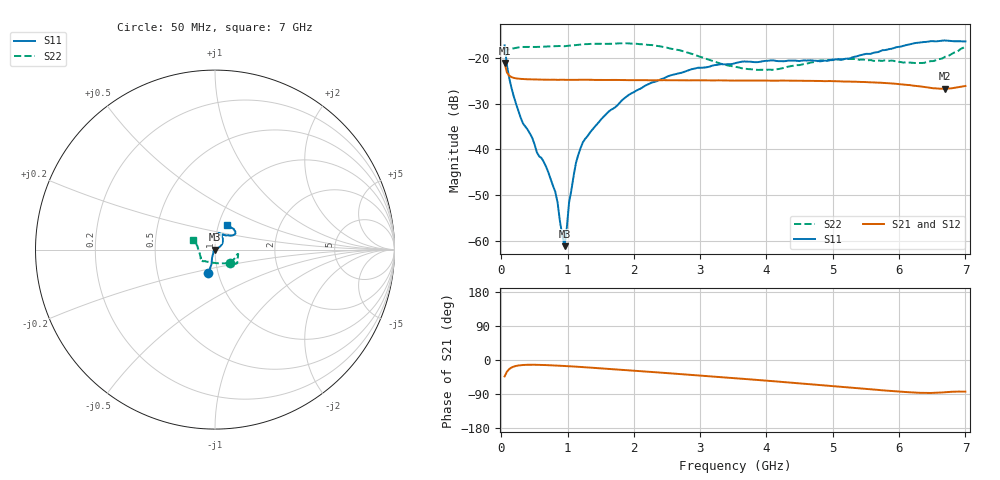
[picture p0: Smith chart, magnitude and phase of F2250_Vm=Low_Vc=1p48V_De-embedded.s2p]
! Integrated Device Technology
! Corporate Headquarters
! 6024 Silver Creek Valley Road
! San Jose, CA 95138  USA
! Phone:  1-408-284-8200
! Toll Free:  1-800-223-1366
! Webpage:  http://www.idt.com/
! Timing and RF Division
! 515 Groton Road, Suite 102
! Westford, MA 01886-6024
! Device:  F2250
! Description: Voltage Variable RF Attenuator
! Frequency:  50.0 -  6000.00 MHz
! Package:  3x3 mm Thin QFN Plastic Package: 16 pin
! Ports:  2 RF, 3 DC
!  Pin  1  = GND
!  Pin  2  = NC
!  Pin  3  = RF1  = Port 1
!  Pin  4  = NC
!  Pin  5  = GND
!  Pin  6  = GND
!  Pin  7  = GND
!  Pin  8  = GND
!  Pin  9  = NC
!  Pin 10  = RF2  = Port 2
!  Pin 11  = NC
!  Pin 12  = GND
!  Pin 13  = GND
!  Pin 14  = VCNTRL
!  Pin 15  = VDD
!  Pin 16  = VMODE
! Vcntrl:  1.480 Volts
! Vmode:  +0.000 Volts
! Vdd:  +3.30  Volts
! Current:  1.192 mA
! Data:  The device was measured on a the F2250 evaluation board which has
!  individual transmission lines to the RF pins.  Data was collected
!  using a calibrated network analyzer.  The evaluation board was
!  de-embedded using a TRL calibration technique.
!  The reference plane is the edge of the package pin.
! Misc:  SN 10
!  Action Tracker AT0258
! Date Measured:  2014-11-26
! Date:  2015-10-15  MJV
! Note:
!  Integrated Device Technology supplies this data as a sample of measured
!  data at the package pin for this product.  Your particular data for this
!  product may vary.
!  Data was taken at 25 degrees C.
!  Integrated Device Technology reserves the right to change this data at anytime.
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# GHz S dB R 50
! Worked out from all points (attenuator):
!   201 points, 50 MHz to 7 GHz, reference 50 ohm
!   highest |S21| = -21.13 dB at 50 MHz (marker M1); lowest = -26.8 dB at 6.687 GHz (marker M2)
!   lowest |S11| = -61.2 dB at 953.5 MHz (marker M3), VSWR 1.00, Z = 49.9 - j0.0709 ohm
!   |S11| at or under -10 dB: start of sweep to end of sweep
!   |S22| runs from -22.6 to -16.8 dB; largest |S21 - S12| = 0.00023
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0.05  -17.26 -105.9  -21.13 -43.3  -21.14 -43.3  -19.12 -42.4
0.1195  -24.43 -106.6  -23.89 -23.9  -23.88 -23.9  -18.10 -15.3
0.29325  -33.12 -115.4  -24.60 -13.7  -24.61 -13.7  -17.62 -11.3
0.6755  -43.79 -138.6  -24.77 -13.4  -24.78 -13.4  -17.50 -15.4
0.8145  -49.28 -173.6  -24.79 -14.5  -24.79 -14.5  -17.45 -18.2
0.9535  -61.18 -125.6  -24.80 -15.8  -24.82 -15.8  -17.46 -20.8
0.98825  -57.12 -16.3  -24.81 -16.1  -24.81 -16.1  -17.39 -21.2
1.023  -51.56 -0.4  -24.80 -16.4  -24.81 -16.4  -17.33 -21.4
1.0925  -45.65 11.3  -24.80 -17.2  -24.81 -17.1  -17.26 -22.5
1.12725  -42.92 15.9  -24.81 -17.5  -24.81 -17.5  -17.19 -23.2
1.2315  -38.45 19.2  -24.78 -18.7  -24.80 -18.7  -17.03 -25.1
1.5095  -33.38 26.5  -24.83 -22.1  -24.82 -22.1  -16.93 -27.8
1.857  -28.83 32.4  -24.86 -26.4  -24.85 -26.4  -16.81 -31.5
2.37825  -24.85 42.1  -24.90 -33.0  -24.89 -33.0  -17.42 -36.3
2.93425  -22.25 56.3  -24.90 -40.2  -24.91 -40.3  -19.43 -46.3
3.525  -21.17 70.1  -24.97 -48.1  -24.96 -48.1  -21.94 -74.5
4.11575  -20.57 78.2  -24.99 -56.1  -24.96 -56.2  -22.58 -111.7
4.7065  -20.60 71.1  -25.04 -64.6  -25.03 -64.7  -20.95 -133.7
5.85325  -18.08 39.1  -25.55 -81.4  -25.56 -81.5  -20.64 -149.7
6.3745  -16.53 40.5  -26.34 -86.9  -26.34 -86.9  -21.09 -170.8
6.68725  -16.19 48.0  -26.77 -85.2  -26.75 -85.2  -19.80 166.9
7  -16.39 62.7  -26.15 -83.4  -26.15 -83.4  -17.52 156.5
